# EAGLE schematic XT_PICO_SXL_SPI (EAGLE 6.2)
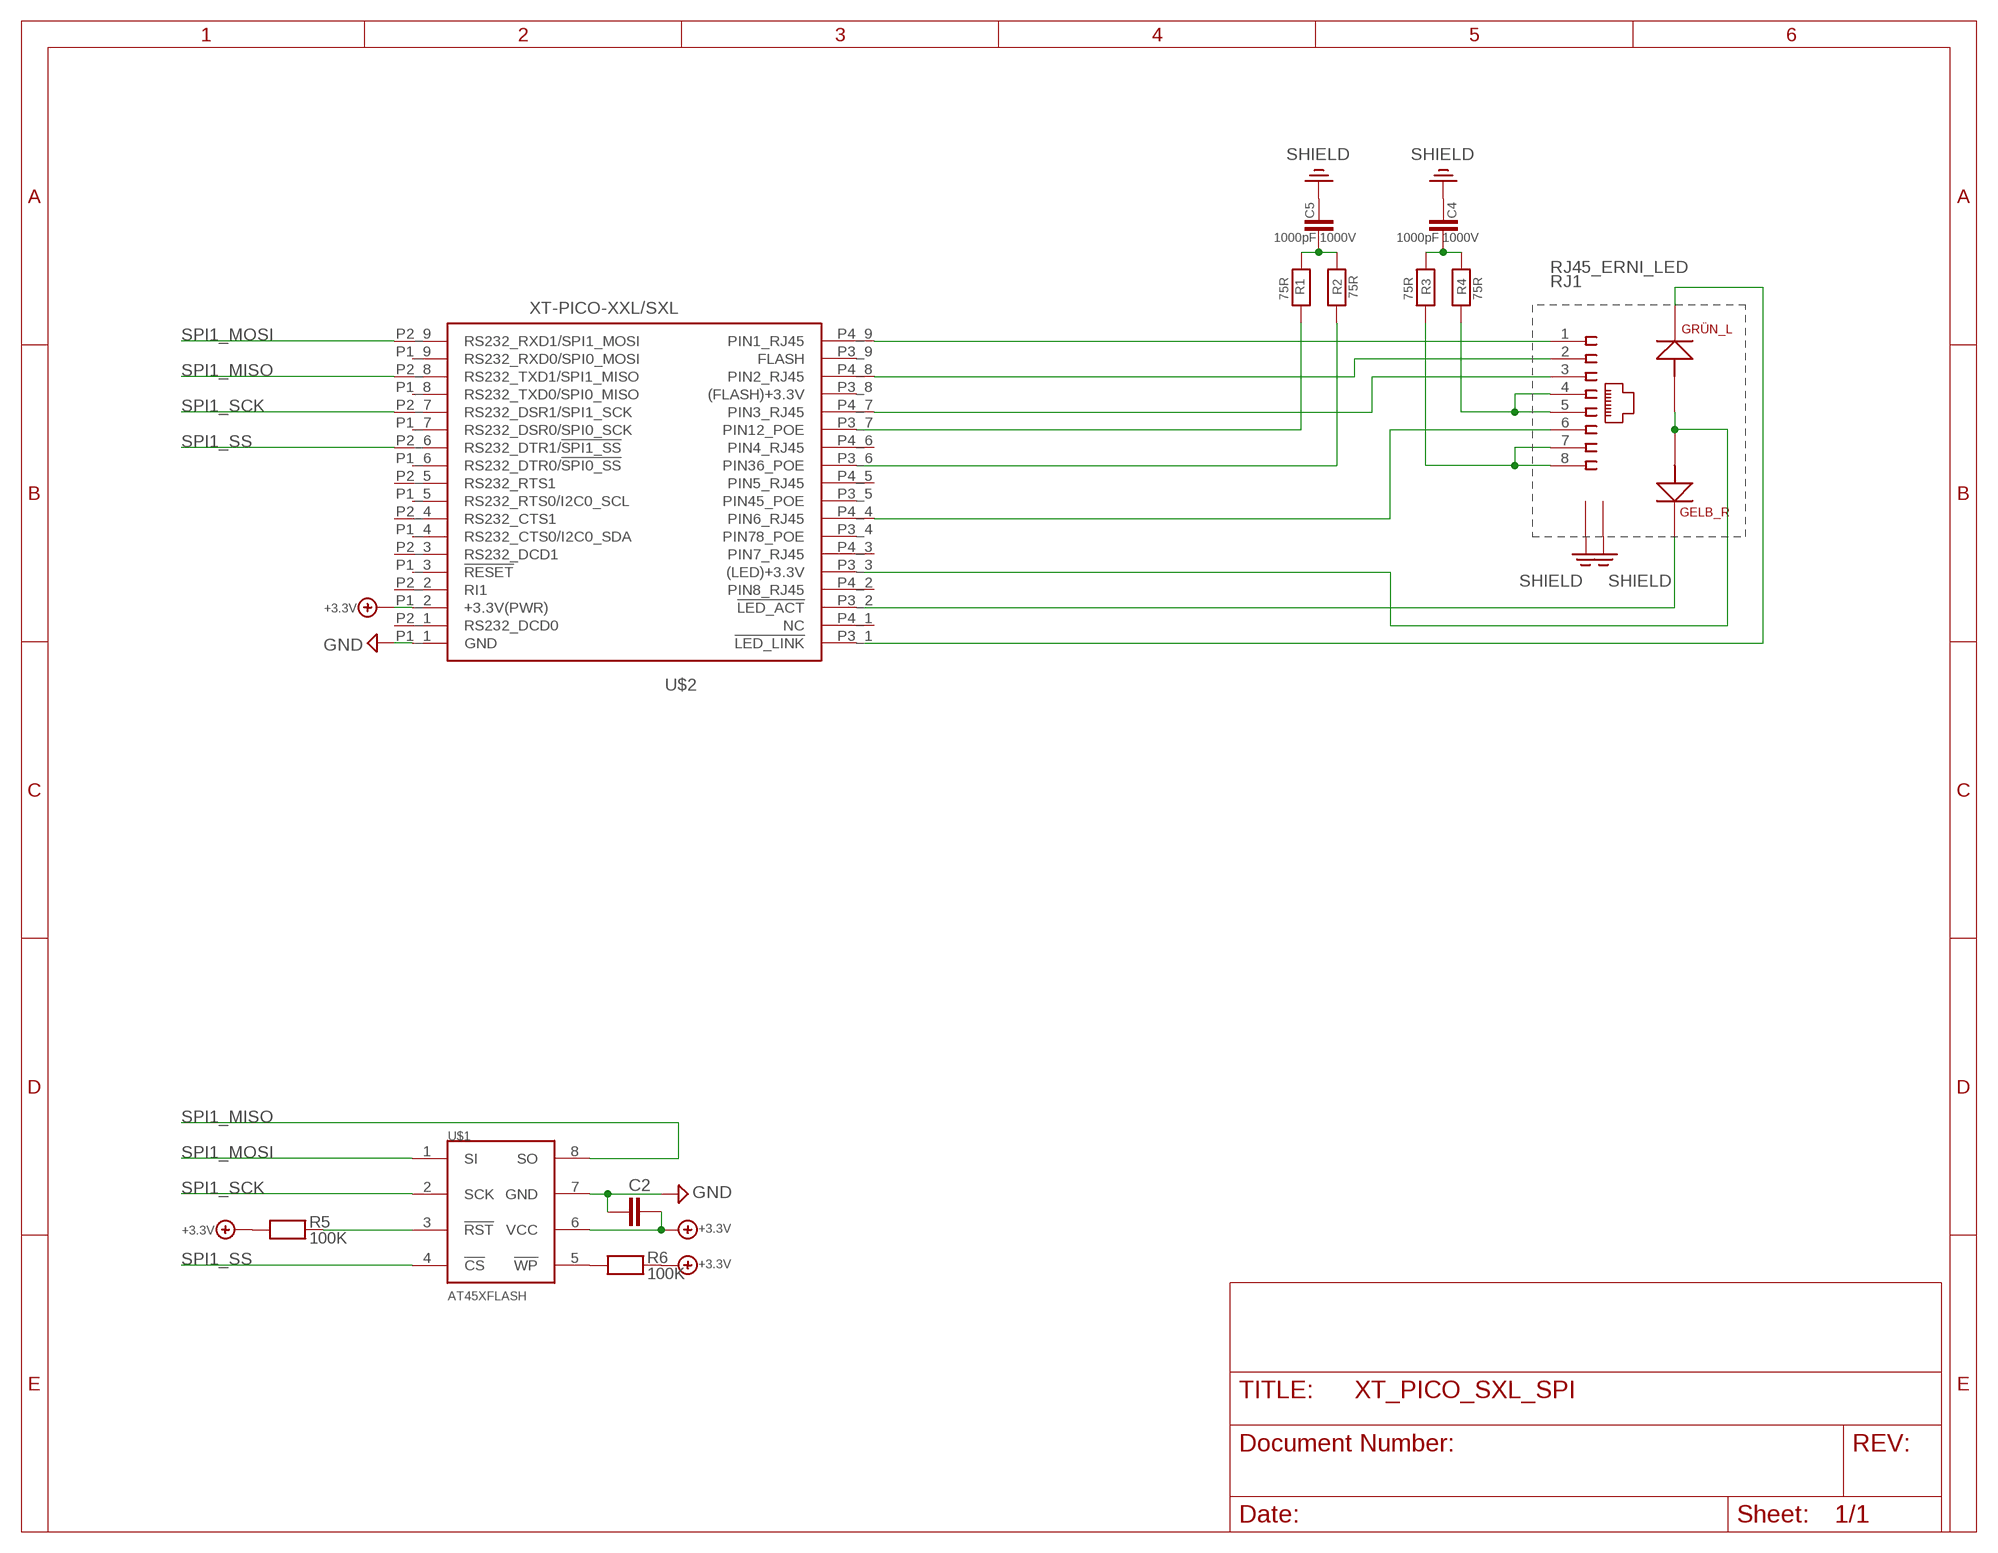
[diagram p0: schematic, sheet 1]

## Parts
C2  CHIP-C-0805  [SMD-0805]
C4  1000pF 1000V  CHIP-C-1210  [SMD-1210]
C5  1000pF 1000V  CHIP-C-1210  [SMD-1210]
R1  75R  CHIP-R-0603  [SMD-0603]
R2  75R  CHIP-R-0603  [SMD-0603]
R3  75R  CHIP-R-0603  [SMD-0603]
R4  75R  CHIP-R-0603  [SMD-0603]
R5  100K  CHIP-R-0603  [SMD-0603]
R6  100K  CHIP-R-0603  [SMD-0603]
RJ1  RJ45_ERNI_LED  [ORCAD_X_ERNI_RJ45_LED]
U$1  AT45XFLASH  [SO-8]
U$2  XT-PICO-XXL/SXL  [XT-PICO-XXL/SXL]

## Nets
+3.3V: C2.2 R5.1 R6.2 U$1.6(VCC) U$2.P1_2(+3.3V(PWR))
GND: C2.1 U$1.7(GND) U$2.P1_1(GND)
N$1: RJ1.1 U$2.P4_9(PIN1_RJ45)
N$2: RJ1.3 U$2.P4_7(PIN3_RJ45)
N$3: R5.2 U$1.3(!RST)
N$4: R1.2 U$2.P3_7(PIN12_POE)
N$5: R6.1 U$1.5(!WP)
N$6: R2.2 U$2.P3_6(PIN36_POE)
N$7: R4.2 RJ1.4 RJ1.5
N$8: RJ1.2 U$2.P4_8(PIN2_RJ45)
N$10: R3.2 RJ1.7 RJ1.8
N$12: RJ1.6 U$2.P4_4(PIN6_RJ45)
N$15: RJ1.A1 RJ1.A2 U$2.P3_3((LED)+3.3V)
N$16: RJ1.K1 U$2.P3_2(!LED_ACT)
N$17: RJ1.K2 U$2.P3_1(!LED_LINK)
N$19: C4.2 R3.1 R4.1
N$20: C5.1 R1.1 R2.1
PE: RJ1.9 RJ1.10 ; supply symbol labelled SHIELD
SHIELD: C4.1 C5.2
SPI1_MISO: U$1.8(SO) U$2.P2_8(RS232_TXD1/SPI1_MISO)
SPI1_MOSI: U$1.1(SI) U$2.P2_9(RS232_RXD1/SPI1_MOSI)
SPI1_SCK: U$1.2(SCK) U$2.P2_7(RS232_DSR1/SPI1_SCK)
SPI1_SS: U$1.4(!CS) U$2.P2_6(RS232_DTR1/!SPI1_SS!)
Unconnected: U$2.P1_3(!RESET) U$2.P1_4(RS232_CTS0/I2C0_SDA) U$2.P1_5(RS232_RTS0/I2C0_SCL) U$2.P1_6(RS232_DTR0/!SPI0_SS!) U$2.P1_7(RS232_DSR0/SPI0_SCK) U$2.P1_8(RS232_TXD0/SPI0_MISO) U$2.P1_9(RS232_RXD0/SPI0_MOSI) U$2.P2_1(RS232_DCD0) U$2.P2_2(RI1) U$2.P2_3(RS232_DCD1) U$2.P2_4(RS232_CTS1) U$2.P2_5(RS232_RTS1) U$2.P3_4(PIN78_POE) U$2.P3_5(PIN45_POE) U$2.P3_8((FLASH)+3.3V) U$2.P3_9(FLASH) U$2.P4_1(NC) U$2.P4_2(PIN8_RJ45) U$2.P4_3(PIN7_RJ45) U$2.P4_5(PIN5_RJ45) U$2.P4_6(PIN4_RJ45)

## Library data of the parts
C2 C4 C5 = XTMACRO:CHIP-C-?: Chip capacitance
R1-R6 = XTMACRO:CHIP-R-?: Chip resistors
RJ1 = XTMACRO:RJ45_ERNI_LED
U$1 = xtnano:AT45XFLASH
U$2 = ak-devices:XT-PICO-XXL/SXL: AK-NORD XT-PICO-XXL/SXL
